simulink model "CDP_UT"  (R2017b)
settings: Solver=FixedStepDiscrete  StartTime=0.0  StopTime=10.0  FixedStep=0.01  RelTol=1e-3  EnableMultiTasking=on
undefined symbols (not defined in the file): ASWTYPE_FALSE, ASWTYPE_TRUE, CaCDP_CellTempNTCVoltTable_mV, CaCDP_CellTempTable_C, CaCDP_CMUPCBTempNTCVoltTable_mV, CaCDP_CMUPCBTempTable_C, CbCDP_DiffBusbarTempStateCheck_flg, CbCDP_DiffCellTempStateCheck_flg, CbCDP_DiffCellVoltStateCheck_flg, CbCDP_IgnorUpdateVld_flg, CbCDP_MaxBusbarTempStateCheck_flg, CbCDP_MaxCellTempStateCheck_flg, CbCDP_MaxCellVoltStateCheck_flg, CbCDP_MinBusbarTempStateCheck_flg, CbCDP_MinCellTempStateCheck_flg, CbCDP_MinCellVoltStateCheck_flg, CcCDP_AFETempConfig_numb, CcCDP_AFETempFltThd_C, CcCDP_AFETempFltThdHys_C, CcCDP_BusbarTempRngFltHiThrd_C, CcCDP_BusbarTempRngFltLowThrd_C, CcCDP_CellDiffFltLevel1_mV, CcCDP_CellDiffFltLevel2_mV, CcCDP_CellDiffFltLevel3_mV, CcCDP_CellTempLowerLimit_C, CcCDP_CellTempRngFltHiThrd_C, CcCDP_CellTempRngFltLowThrd_C, CcCDP_CellTempUpperLimit_C, CcCDP_CellVoltConfig_numb, CcCDP_CellVoltLowerLimit_mV, CcCDP_CellVoltRngHiThrd_mV, CcCDP_CellVoltRngLowThrd_mV, CcCDP_CellVoltUpdateThrd_numb, CcCDP_CellVoltUpperLimit_mV, CcCDP_ChrgMaxCellTempFltLv1Thrd_C, CcCDP_ChrgMaxCellTempFltLv2Thrd_C, CcCDP_ChrgMaxCellTempFltLv3Thrd_C, CcCDP_ChrgMaxCellTempReturnDiff_C, CcCDP_ChrgMinCellTempFltLv1Thrd_C, CcCDP_ChrgMinCellTempFltLv2Thrd_C, CcCDP_ChrgMinCellTempFltLv3Thrd_C, CcCDP_ChrgMinCellTempReturnDiff_C, CcCDP_CMUPCBTempConfig_numb, CcCDP_CMUPCBTempFltThd_C, CcCDP_CMUPCBTempFltThdHys_C, CcCDP_DiffBusbarTempFltLevel1Thrd_C, CcCDP_DiffBusbarTempFltLevel2Thrd_C, CcCDP_DiffBusbarTempReturnDifference_C, CcCDP_DiffCellTempFltLevel1Thrd_C, CcCDP_DiffCellTempFltLevel2Thrd_C, CcCDP_DiffCellTempReturnDifference_C, CcCDP_DiffCellVoltReturnDifference_mV, CcCDP_DiffVoltCheckMaxCellTempCondition_C, CcCDP_DiffVoltCheckMaxCellVoltCondition_mV, CcCDP_DiffVoltCheckMinCellTempCondition_C, CcCDP_DiffVoltCheckMinCellVoltCondition_mV, CcCDP_DiffVoltCheckPackCurrCondition_A, CcCDP_MaxAFETempIniVal_C, CcCDP_MaxBusbarTempFltLevel1Thrd_C, CcCDP_MaxBusbarTempFltLevel2Thrd_C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
libraries: AIWAYS_Powertrain_BMS_lib x148, simulink x8
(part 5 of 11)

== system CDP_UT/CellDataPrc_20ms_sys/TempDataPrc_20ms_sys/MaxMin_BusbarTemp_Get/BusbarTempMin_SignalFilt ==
  GeUDS_CapSel_enum : Inport
  LbCDP_AnyBusbarTempVld_flg : Inport  Port=2
  LcCDP_MinBusbarTemp_C : Inport  Port=3
  LcCDP_MinBusbarTempNumb_numb : Inport  Port=4
  1D_Config_Word : AIWAYS_Powertrain_BMS_lib/Signals/1D_Config_Word  Default_CalPar_Name=CcCDP_CATL203MaxCellTempFilCfig_numb  CATL153Ah_CalPar_Name=CcCDP_CATL177MaxCellTempFilCfig_numb  CATL180Ah_CalPar_Name=CcCDP_CATL177MaxCellTempFilCfig_numb  CATL177Ah_CalPar_Name=CcCDP_CATL177MaxCellTempFilCfig_numb  CATL203Ah_CalPar_Name=CcCDP_CATL203MaxCellTempFilCfig_numb  CATL51Ah_CalPar_Name=CcCDP_CATL177MaxCellTempFilCfig_numb  CATL132Ah_CalPar_Name=CcCDP_CATL177MaxCellTempFilCfig_numb  XWD75Ah_CalPar_Name=CcCDP_CATL177MaxCellTempFilCfig_numb  TFE177Ah_CalPar_Name=CcCDP_CATL177MaxCellTempFilCfig_numb  CATLCTP248Ah_CalPar_Name=CcCDP_CATL177MaxCellTempFilCfig_numb
  InputValueCalc : Stateflow chart  TreatAsAtomicUnit=on
  MaxValue_sort : Stateflow chart  TreatAsAtomicUnit=on
  SignalDelay1 : Subsystem  Commented=on
  Unit Delay21 : UnitDelay  SampleTime=-1  StateName=StateName
  ValueCalc : Subsystem
  ValueIndexCalc : Subsystem
  GcCDP_MinBusbarTemp_C : Outport
  GcCDP_MinBusbarTempNumb_numb : Outport  Port=2
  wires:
  LbCDP_AnyBusbarTempVld_flg/1 -> InputValueCalc/2(Rige), ValueIndexCalc/3(LbCDP_AnyBusbarTempVld_flg)
  GeUDS_CapSel_enum/1 -> 1D_Config_Word/1
  InputValueCalc/1(Output_Value) -> Unit Delay21/1, MaxValue_sort/1(Input_Value)
  1D_Config_Word/1 -> ValueCalc/3(CcCDP_CellTempFilConfig_numb), MaxValue_sort/2(Input_dim)
  ValueCalc/1(GcCDP_MinBusbarTemp_C) -> GcCDP_MinBusbarTemp_C/1
  ValueIndexCalc/1(GcCDP_MinBusbarTempNumb_numb) -> GcCDP_MinBusbarTempNumb_numb/1
  LcCDP_MinBusbarTempNumb_numb/1 -> ValueIndexCalc/2(LcCDP_MinBusbarTempNumb_numb)
  LcCDP_MinBusbarTemp_C/1 -> InputValueCalc/1(Input_Value)
  Unit Delay21/1 -> InputValueCalc/3(Old_Value)
  MaxValue_sort/1(Output_Value) -> ValueCalc/1(Output_Value)
  MaxValue_sort/2(Output_index) -> ValueCalc/2(Output_index)
  ValueCalc/2(Output_index1) -> ValueIndexCalc/1(Output_index1)

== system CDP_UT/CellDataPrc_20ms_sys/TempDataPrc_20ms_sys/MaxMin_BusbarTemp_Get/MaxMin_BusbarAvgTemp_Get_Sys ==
  LaCDP_BusbarTemp_C : Inport
  GcUDS_BusbarTempNumb_numb : Inport  Port=2
  Enable : EnablePort  StatesWhenEnabling=reset
  Divide1 : Product  Inputs=*/  OutDataTypeStr=single
  MinBusbarTemp_ForIterator : Subsystem  TreatAsAtomicUnit=on
  OverWrite1 : AIWAYS_Powertrain_BMS_lib/Signals/OverWrite  OverWrite_Value=CcCDP_AvgBusbarTempOvr_C  OverWrite_flag=CbCDP_AvgBusbarTempOvrSwt_flg
  GcCDP_AvgBusbarTemp_C : Outport
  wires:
  GcUDS_BusbarTempNumb_numb/1 -> Divide1/2, MinBusbarTemp_ForIterator/2(GcUDS_BusbarTempNumb_numb)
  MinBusbarTemp_ForIterator/1(LcCDP_SumBusbarTemp_C) -> Divide1/1
  Divide1/1 -> OverWrite1/1
  OverWrite1/1 -> GcCDP_AvgBusbarTemp_C/1  "GcCDP_AvgBusbarTemp_C"
  LaCDP_BusbarTemp_C/1 -> MinBusbarTemp_ForIterator/1(LaCDP_BusbarTemp_C)

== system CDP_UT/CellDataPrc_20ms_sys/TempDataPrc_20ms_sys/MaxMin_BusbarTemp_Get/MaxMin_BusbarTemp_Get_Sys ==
  LaCDP_BusbarTempVld_flg : Inport
  LaCDP_BusbarTemp_C : Inport  Port=2
  GcUDS_BusbarTempNumb_numb : Inport  Port=3
  GaISP_BusbarTempUpdCnt_numb : Inport  Port=4
  Enable : EnablePort  StatesWhenEnabling=reset
  Comparison4 : RelationalOperator  Operator===  OutDataTypeStr=boolean
  Constant1 : Constant  Value=CDP_CONST0_NUMB
  Constant2 : Constant  Value=CbCDP_IgnorUpdateVld_flg
  Logical : Logic  OutDataTypeStr=boolean
  MinBusbarTemp_ForIterator : Subsystem  TreatAsAtomicUnit=on
  Switch : Switch  Criteria=u2 ~= 0  Threshold=1  RndMeth=Zero
  LcCDP_MaxBusbarTemp_C : Outport
  LcCDP_MaxBusbarTempNumb_numb : Outport  Port=2
  LcCDP_MinBusbarTemp_C : Outport  Port=3
  LcCDP_MinBusbarTempNumb_numb : Outport  Port=4
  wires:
  MinBusbarTemp_ForIterator/3(LcCDP_MaxBusbarTempNumb_numb) -> LcCDP_MaxBusbarTempNumb_numb/1  "LcCDP_MaxBusbarTempNumb_numb"
  MinBusbarTemp_ForIterator/4(LcCDP_MaxBusbarTemp_C) -> LcCDP_MaxBusbarTemp_C/1  "LcCDP_MaxBusbarTemp_C"
  MinBusbarTemp_ForIterator/1(LcCDP_MinBusbarTemp_C) -> LcCDP_MinBusbarTemp_C/1  "LcCDP_MinBusbarTemp_C"
  MinBusbarTemp_ForIterator/2(LcCDP_MinBusbarTempNumb_numb) -> LcCDP_MinBusbarTempNumb_numb/1  "LcCDP_MinBusbarTempNumb_numb"
  LaCDP_BusbarTemp_C/1 -> MinBusbarTemp_ForIterator/1(LaCDP_BusbarTemp_C)
  GcUDS_BusbarTempNumb_numb/1 -> MinBusbarTemp_ForIterator/3(GcUDS_BusbarTempNumb_numb)
  Comparison4/1 -> Logical/2
  GaISP_BusbarTempUpdCnt_numb/1 -> Comparison4/1
  LaCDP_BusbarTempVld_flg/1 -> Logical/1, Switch/1
  Logical/1 -> Switch/3
  Constant1/1 -> Comparison4/2
  Constant2/1 -> Switch/2
  Switch/1 -> MinBusbarTemp_ForIterator/2(LaCDP_BusbarTempVld_flg)

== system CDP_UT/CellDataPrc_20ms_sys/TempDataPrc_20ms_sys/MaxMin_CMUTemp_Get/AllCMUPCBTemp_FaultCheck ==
  GaCDP_CMUPCBTempVld_flg : Inport
  CMUTempVld : Subsystem
  Constant4 : Constant  Value=CcCDP_CMUPCBTempConfig_numb
  LbCDP_AnyCMUTempVld_flg : Outport
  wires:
  GaCDP_CMUPCBTempVld_flg/1 -> CMUTempVld/1(GaCDP_CMUPCBTempVld_flg)
  Constant4/1 -> CMUTempVld/2(CcCDP_CMUTempConfig_numb)
  CMUTempVld/1(LbCDP_AnyCMUTempVld_flg) -> LbCDP_AnyCMUTempVld_flg/1

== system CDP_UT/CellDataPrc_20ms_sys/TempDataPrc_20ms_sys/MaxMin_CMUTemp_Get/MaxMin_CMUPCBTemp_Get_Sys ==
  GaCDP_CMUPCBTempVld_flg : Inport
  GaCDP_CMUPCBTemp_C : Inport  Port=2
  Enable : EnablePort  StatesWhenEnabling=reset
  CDP_GcCDP_MaxCMUPCBTempNumb_numb : AIWAYS_Powertrain_BMS_lib/Signals/OverWrite  OverWrite_Value=CcCDP_MaxCMUPCBTempNumbOvr_numb  OverWrite_flag=CbCDP_MaxCMUPCBTempNumbOvrSwt_flg
  CDP_GcCDP_MaxCMUPCBTemp_C : AIWAYS_Powertrain_BMS_lib/Signals/OverWrite  OverWrite_Value=CcCDP_MaxCMUPCBTempOvr_C  OverWrite_flag=CbCDP_MaxCMUPCBTempOvrSwt_flg
  CDP_GcCDP_MinCMUPCBTempNumb_numb : AIWAYS_Powertrain_BMS_lib/Signals/OverWrite  OverWrite_Value=CcCDP_MinCMUPCBTempNumbOvr_numb  OverWrite_flag=CbCDP_MinCMUPCBTempNumbOvrSwt_flg
  CDP_GcCDP_MinCMUPCBTemp_C : AIWAYS_Powertrain_BMS_lib/Signals/OverWrite  OverWrite_Value=CcCDP_MinCMUPCBTempOvr_C  OverWrite_flag=CbCDP_MinCMUPCBTempOvrSwt_flg
  Constant3 : Constant  Value=CcCDP_CMUPCBTempConfig_numb
  MinCMUTemp_ForIterator : Subsystem  TreatAsAtomicUnit=on
  GcCDP_MaxCMUPCBTemp_C : Outport
  GcCDP_MaxCMUPCBTempNumb_numb : Outport  Port=2
  GcCDP_MinCMUPCBTemp_C : Outport  Port=3
  GcCDP_MinCMUPCBTempNumb_numb : Outport  Port=4
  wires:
  Constant3/1 -> MinCMUTemp_ForIterator/3(CcCDP_CMUPCBTempConfig_numb)  "CcCDP_CMUPCBTempConfig_numb"
  GaCDP_CMUPCBTemp_C/1 -> MinCMUTemp_ForIterator/1(GaCDP_CMUPCBTemp_C)
  MinCMUTemp_ForIterator/1(LcCDP_MinCMUPCBTemp_C) -> CDP_GcCDP_MinCMUPCBTemp_C/1
  MinCMUTemp_ForIterator/2(LcCDP_MinCMUPCBTempNumb_numb) -> CDP_GcCDP_MinCMUPCBTempNumb_numb/1
  GaCDP_CMUPCBTempVld_flg/1 -> MinCMUTemp_ForIterator/2(GaCDP_CMUPCBTempVld_flg)
  CDP_GcCDP_MinCMUPCBTempNumb_numb/1 -> GcCDP_MinCMUPCBTempNumb_numb/1  "GcCDP_MinCMUPCBTempNumb_numb"
  CDP_GcCDP_MinCMUPCBTemp_C/1 -> GcCDP_MinCMUPCBTemp_C/1  "GcCDP_MinCMUPCBTemp_C"
  CDP_GcCDP_MaxCMUPCBTempNumb_numb/1 -> GcCDP_MaxCMUPCBTempNumb_numb/1  "GcCDP_MaxCMUPCBTempNumb_numb"
  CDP_GcCDP_MaxCMUPCBTemp_C/1 -> GcCDP_MaxCMUPCBTemp_C/1  "GcCDP_MaxCMUPCBTemp_C"
  MinCMUTemp_ForIterator/3(LcCDP_MaxCMUPCBTempNumb_numb) -> CDP_GcCDP_MaxCMUPCBTempNumb_numb/1
  MinCMUTemp_ForIterator/4(LcCDP_MaxCMUPCBTemp_C) -> CDP_GcCDP_MaxCMUPCBTemp_C/1

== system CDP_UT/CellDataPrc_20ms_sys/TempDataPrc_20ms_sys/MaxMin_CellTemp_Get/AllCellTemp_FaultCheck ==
  GaCDP_CellTempVld_flg : Inport
  GcUDS_CellTempNumb_numb : Inport  Port=2
  GaISP_CellTempUpdCnt_numb : Inport  Port=3
  CellTempVld : Subsystem
  Comparison4 : RelationalOperator  Operator===  OutDataTypeStr=boolean
  Constant1 : Constant  Value=CDP_CONST0_NUMB
  Constant2 : Constant  Value=CbCDP_IgnorUpdateVld_flg
  Logical : Logic  OutDataTypeStr=boolean
  OverWrite : AIWAYS_Powertrain_BMS_lib/Signals/OverWrite  OverWrite_Value=CbCDP_AllCellTempVldOvr_flg  OverWrite_flag=CbCDP_AllCellTempVldOvrSwt_flg
  Switch : Switch  Criteria=u2 ~= 0  Threshold=1  RndMeth=Zero
  GbCDP_AllCellTempVld_flg : Outport
  LbCDP_AnyCellTempVld_flg : Outport  Port=2
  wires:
  CellTempVld/1(LbCDP_CellTempVld_flg) -> OverWrite/1
  OverWrite/1 -> GbCDP_AllCellTempVld_flg/1  "GbCDP_AllCellTempVld_flg"
  GcUDS_CellTempNumb_numb/1 -> CellTempVld/2(GcUDS_CellTempNumb_numb)
  CellTempVld/2(LbCDP_AnyCellTempVld_flg) -> LbCDP_AnyCellTempVld_flg/1
  Switch/1 -> CellTempVld/1(GaCDP_CellTempVld_flg)
  GaCDP_CellTempVld_flg/1 -> Switch/1, Logical/1
  GaISP_CellTempUpdCnt_numb/1 -> Comparison4/1
  Constant2/1 -> Switch/2
  Constant1/1 -> Comparison4/2
  Logical/1 -> Switch/3
  Comparison4/1 -> Logical/2

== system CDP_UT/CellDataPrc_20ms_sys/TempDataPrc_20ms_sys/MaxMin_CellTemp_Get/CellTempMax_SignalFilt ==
  LcCDP_MaxCellTemp_C : Inport
  LcCDP_MaxCellTempNumb_numb : Inport  Port=2
  LbCDP_AnyCellTempVld_flg : Inport  Port=3
  GeUDS_CapSel_enum : Inport  Port=4
  1D_Config_Word : AIWAYS_Powertrain_BMS_lib/Signals/1D_Config_Word  Default_CalPar_Name=CcCDP_CATL203MaxCellTempFilCfig_numb  CATL153Ah_CalPar_Name=CcCDP_CATL177MaxCellTempFilCfig_numb  CATL180Ah_CalPar_Name=CcCDP_CATL177MaxCellTempFilCfig_numb  CATL177Ah_CalPar_Name=CcCDP_CATL177MaxCellTempFilCfig_numb  CATL203Ah_CalPar_Name=CcCDP_CATL203MaxCellTempFilCfig_numb  CATL51Ah_CalPar_Name=CcCDP_CATL177MaxCellTempFilCfig_numb  CATL132Ah_CalPar_Name=CcCDP_CATL177MaxCellTempFilCfig_numb  XWD75Ah_CalPar_Name=CcCDP_CATL177MaxCellTempFilCfig_numb  TFE177Ah_CalPar_Name=CcCDP_CATL177MaxCellTempFilCfig_numb  CATLCTP248Ah_CalPar_Name=CcCDP_CATL177MaxCellTempFilCfig_numb
  InputValueCalc : Stateflow chart  TreatAsAtomicUnit=on
  MaxValue_sort : Stateflow chart  TreatAsAtomicUnit=on
  SignalDelay1 : Subsystem  Commented=on
  Unit Delay21 : UnitDelay  SampleTime=-1  StateName=StateName
  ValueCalc : Subsystem
  ValueIndexCalc : Subsystem
  GcCDP_MaxCellTemp_C : Outport
  GcCDP_MaxCellTempNumb_numb : Outport  Port=2
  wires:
  ValueCalc/2(Output_index1) -> ValueIndexCalc/1(Output_index1)
  MaxValue_sort/2(Output_index) -> ValueCalc/2(Output_index)
  MaxValue_sort/1(Output_Value) -> ValueCalc/1(Output_Value)
  Unit Delay21/1 -> InputValueCalc/3(Old_Value)
  LcCDP_MaxCellTemp_C/1 -> InputValueCalc/1(Input_Value)
  LcCDP_MaxCellTempNumb_numb/1 -> ValueIndexCalc/2(LcCDP_MaxCellTempNumb_numb)
  ValueIndexCalc/1(GcCDP_MaxCellTempNumb_numb) -> GcCDP_MaxCellTempNumb_numb/1
  ValueCalc/1(GcCDP_MaxCellTemp_C) -> GcCDP_MaxCellTemp_C/1
  1D_Config_Word/1 -> MaxValue_sort/2(Input_dim), ValueCalc/3(CcCDP_CellTempFilConfig_numb)
  InputValueCalc/1(Output_Value) -> MaxValue_sort/1(Input_Value), Unit Delay21/1
  GeUDS_CapSel_enum/1 -> 1D_Config_Word/1
  LbCDP_AnyCellTempVld_flg/1 -> ValueIndexCalc/3(LbCDP_AnyCellTempVld_flg), InputValueCalc/2(Rige)

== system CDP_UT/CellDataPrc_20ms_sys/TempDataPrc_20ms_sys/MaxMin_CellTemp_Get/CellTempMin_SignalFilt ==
  GeUDS_CapSel_enum : Inport
  LbCDP_AnyCellTempVld_flg : Inport  Port=2
  LcCDP_MinCellTemp_C : Inport  Port=3
  LcCDP_MinCellTempNumb_numb : Inport  Port=4
  1D_Config_Word : AIWAYS_Powertrain_BMS_lib/Signals/1D_Config_Word  Default_CalPar_Name=CcCDP_CATL203MaxCellTempFilCfig_numb  CATL153Ah_CalPar_Name=CcCDP_CATL177MaxCellTempFilCfig_numb  CATL180Ah_CalPar_Name=CcCDP_CATL177MaxCellTempFilCfig_numb  CATL177Ah_CalPar_Name=CcCDP_CATL177MaxCellTempFilCfig_numb  CATL203Ah_CalPar_Name=CcCDP_CATL203MaxCellTempFilCfig_numb  CATL51Ah_CalPar_Name=CcCDP_CATL177MaxCellTempFilCfig_numb  CATL132Ah_CalPar_Name=CcCDP_CATL177MaxCellTempFilCfig_numb  XWD75Ah_CalPar_Name=CcCDP_CATL177MaxCellTempFilCfig_numb  TFE177Ah_CalPar_Name=CcCDP_CATL177MaxCellTempFilCfig_numb  CATLCTP248Ah_CalPar_Name=CcCDP_CATL177MaxCellTempFilCfig_numb
  InputValueCalc : Stateflow chart  TreatAsAtomicUnit=on
  MaxValue_sort : Stateflow chart  TreatAsAtomicUnit=on
  SignalDelay1 : Subsystem  Commented=on
  Unit Delay21 : UnitDelay  SampleTime=-1  StateName=StateName
  ValueCalc : Subsystem
  ValueIndexCalc : Subsystem
  GcCDP_MinCellTemp_C : Outport
  GcCDP_MinCellTempNumb_numb : Outport  Port=2
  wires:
  LbCDP_AnyCellTempVld_flg/1 -> InputValueCalc/2(Rige), ValueIndexCalc/3(LbCDP_AnyCellTempVld_flg)
  GeUDS_CapSel_enum/1 -> 1D_Config_Word/1
  InputValueCalc/1(Output_Value) -> Unit Delay21/1, MaxValue_sort/1(Input_Value)
  1D_Config_Word/1 -> ValueCalc/3(CcCDP_CellTempFilConfig_numb), MaxValue_sort/2(Input_dim)
  ValueCalc/1(GcCDP_MinCellTemp_C) -> GcCDP_MinCellTemp_C/1
  ValueIndexCalc/1(GcCDP_MinCellTempNumb_numb) -> GcCDP_MinCellTempNumb_numb/1
  LcCDP_MinCellTempNumb_numb/1 -> ValueIndexCalc/2(LcCDP_MinCellTempNumb_numb)
  LcCDP_MinCellTemp_C/1 -> InputValueCalc/1(Input_Value)
  Unit Delay21/1 -> InputValueCalc/3(Old_Value)
  MaxValue_sort/1(Output_Value) -> ValueCalc/1(Output_Value)
  MaxValue_sort/2(Output_index) -> ValueCalc/2(Output_index)
  ValueCalc/2(Output_index1) -> ValueIndexCalc/1(Output_index1)

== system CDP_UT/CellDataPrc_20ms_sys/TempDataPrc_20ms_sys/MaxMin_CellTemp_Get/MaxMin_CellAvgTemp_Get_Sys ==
  LaCDP_CellTemp_C : Inport
  GcUDS_CellTempNumb_numb : Inport  Port=2
  Enable : EnablePort  StatesWhenEnabling=reset
  Divide1 : Product  Inputs=*/  OutDataTypeStr=single
  MinCellTemp_ForIterator : Subsystem  TreatAsAtomicUnit=on
  OverWrite1 : AIWAYS_Powertrain_BMS_lib/Signals/OverWrite  OverWrite_Value=CcCDP_AvgCellTempOvr_C  OverWrite_flag=CbCDP_AvgCellTempOvrSwt_flg
  GcCDP_AvgCellTemp_C : Outport
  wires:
  LaCDP_CellTemp_C/1 -> MinCellTemp_ForIterator/1(LaCDP_CellTemp_C)
  OverWrite1/1 -> GcCDP_AvgCellTemp_C/1  "GcCDP_AvgCellTemp_C"
  Divide1/1 -> OverWrite1/1
  MinCellTemp_ForIterator/1(LcCDP_SumCellTemp_C) -> Divide1/1
  GcUDS_CellTempNumb_numb/1 -> MinCellTemp_ForIterator/2(GcUDS_CellTempNumb_numb), Divide1/2

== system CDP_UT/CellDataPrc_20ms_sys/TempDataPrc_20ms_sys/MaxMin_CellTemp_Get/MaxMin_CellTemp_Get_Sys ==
  GaCDP_CellTempVld_flg : Inport
  LaCDP_CellTemp_C : Inport  Port=2
  GcUDS_CellTempNumb_numb : Inport  Port=3
  GaISP_CellTempUpdCnt_numb : Inport  Port=4
  Enable : EnablePort  StatesWhenEnabling=reset
  Comparison4 : RelationalOperator  Operator===  OutDataTypeStr=boolean
  Constant1 : Constant  Value=CDP_CONST0_NUMB
  Constant2 : Constant  Value=CbCDP_IgnorUpdateVld_flg
  Logical : Logic  OutDataTypeStr=boolean
  MinCellTemp_ForIterator : Subsystem  TreatAsAtomicUnit=on
  Switch : Switch  Criteria=u2 ~= 0  Threshold=1  RndMeth=Zero
  LcCDP_MaxCellTemp_C : Outport
  LcCDP_MaxCellTempNumb_numb : Outport  Port=2
  LcCDP_MinCellTemp_C : Outport  Port=3
  LcCDP_MinCellTempNumb_numb : Outport  Port=4
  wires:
  MinCellTemp_ForIterator/1(LcCDP_MinCellTemp_C) -> LcCDP_MinCellTemp_C/1  "LcCDP_MinCellTemp_C"
  MinCellTemp_ForIterator/2(LcCDP_MinCellTempNumb_numb) -> LcCDP_MinCellTempNumb_numb/1  "LcCDP_MinCellTempNumb_numb"
  MinCellTemp_ForIterator/3(LcCDP_MaxCellTempNumb_numb) -> LcCDP_MaxCellTempNumb_numb/1  "LcCDP_MaxCellTempNumb_numb"
  MinCellTemp_ForIterator/4(LcCDP_MaxCellTemp_C) -> LcCDP_MaxCellTemp_C/1  "LcCDP_MaxCellTemp_C"
  GcUDS_CellTempNumb_numb/1 -> MinCellTemp_ForIterator/3(GcUDS_CellTempNumb_numb)
  GaCDP_CellTempVld_flg/1 -> Switch/1, Logical/1
  Comparison4/1 -> Logical/2
  Logical/1 -> Switch/3
  Constant1/1 -> Comparison4/2
  GaISP_CellTempUpdCnt_numb/1 -> Comparison4/1
  Constant2/1 -> Switch/2
  LaCDP_CellTemp_C/1 -> MinCellTemp_ForIterator/1(LaCDP_CellTemp_C)
  Switch/1 -> MinCellTemp_ForIterator/2(GaCDP_CellTempVld_flg)

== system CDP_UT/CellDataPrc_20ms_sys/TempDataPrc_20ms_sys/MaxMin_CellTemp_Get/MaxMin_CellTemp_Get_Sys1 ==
  GaCDP_CellTempVld_flg : Inport
  GaCDP_CellTemp_C : Inport  Port=2
  GcUDS_CellTempNumb_numb : Inport  Port=3
  Enable : EnablePort  StatesWhenEnabling=reset
  MinCellTemp_ForIterator : Subsystem  TreatAsAtomicUnit=on
  OverWrite : AIWAYS_Powertrain_BMS_lib/Signals/OverWrite  OverWrite_Value=CcCDP_MinCellTempOvr_C  OverWrite_flag=CbCDP_MinCellTempOvrSwt_flg
  OverWrite1 : AIWAYS_Powertrain_BMS_lib/Signals/OverWrite  OverWrite_Value=CcCDP_MinCellTempNumbOvr_numb  OverWrite_flag=CbCDP_MinCellTempNumbOvrSwt_flg
  OverWrite2 : AIWAYS_Powertrain_BMS_lib/Signals/OverWrite  OverWrite_Value=CcCDP_MaxCellTempOvr_C  OverWrite_flag=CbCDP_MaxCellTempOvrSwt_flg
  OverWrite3 : AIWAYS_Powertrain_BMS_lib/Signals/OverWrite  OverWrite_Value=CcCDP_MaxCellTempNumbOvr_numb  OverWrite_flag=CbCDP_MaxCellTempNumbOvrSwt_flg
  GcCDP_MaxCellTemp_C : Outport
  GcCDP_MaxCellTempNumb_numb : Outport  Port=2
  GcCDP_MinCellTemp_C : Outport  Port=3
  GcCDP_MinCellTempNumb_numb : Outport  Port=4
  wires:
  GaCDP_CellTemp_C/1 -> MinCellTemp_ForIterator/1(GaCDP_CellTemp_C)
  OverWrite1/1 -> GcCDP_MinCellTempNumb_numb/1  "GcCDP_MinCellTempNumb_numb"
  OverWrite/1 -> GcCDP_MinCellTemp_C/1  "GcCDP_MinCellTemp_C"
  OverWrite2/1 -> GcCDP_MaxCellTemp_C/1  "GcCDP_MaxCellTemp_C"
  OverWrite3/1 -> GcCDP_MaxCellTempNumb_numb/1  "GcCDP_MaxCellTempNumb_numb"
  MinCellTemp_ForIterator/1(LcCDP_MinCellTemp_C) -> OverWrite/1
  MinCellTemp_ForIterator/2(LcCDP_MinCellTempNumb_numb) -> OverWrite1/1
  MinCellTemp_ForIterator/3(LcCDP_MaxCellTempNumb_numb) -> OverWrite3/1
  MinCellTemp_ForIterator/4(LcCDP_MaxCellTemp_C) -> OverWrite2/1
  GaCDP_CellTempVld_flg/1 -> MinCellTemp_ForIterator/2(GaCDP_CellTempVld_flg)
  GcUDS_CellTempNumb_numb/1 -> MinCellTemp_ForIterator/3(GcUDS_CellTempNumb_numb)

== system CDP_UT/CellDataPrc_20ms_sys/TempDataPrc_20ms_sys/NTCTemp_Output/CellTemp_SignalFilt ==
  GcUDS_CellTempNumb_numb : Inport
  GeUDS_CapSel_enum : Inport  Port=2
  LaCDP_CellTempUpdateVld_flg : Inport  Port=3
  LaCDP_CellTemp_C : Inport  Port=4
  1D_Config_Word : AIWAYS_Powertrain_BMS_lib/Signals/1D_Config_Word  Default_CalPar_Name=CcCDP_CATL203CellTempFilCfig_numb  CATL153Ah_CalPar_Name=CcCDP_CATL177CellTempFilCfig_numb  CATL180Ah_CalPar_Name=CcCDP_CATL177CellTempFilCfig_numb  CATL177Ah_CalPar_Name=CcCDP_CATL177CellTempFilCfig_numb  CATL203Ah_CalPar_Name=CcCDP_CATL203CellTempFilCfig_numb  CATL51Ah_CalPar_Name=CcCDP_CATL177CellTempFilCfig_numb  CATL132Ah_CalPar_Name=CcCDP_CATL177CellTempFilCfig_numb  XWD75Ah_CalPar_Name=CcCDP_CATL177CellTempFilCfig_numb  TFE177Ah_CalPar_Name=CcCDP_CATL177CellTempFilCfig_numb  CATLCTP248Ah_CalPar_Name=CcCDP_CATL177CellTempFilCfig_numb
  Comparison1 : RelationalOperator  Operator===  OutDataTypeStr=boolean
  Constant6 : Constant  Value=ASWTYPE_FALSE
  InputValueCalc : Stateflow chart  TreatAsAtomicUnit=on
  MaxValue_sort : Stateflow chart  TreatAsAtomicUnit=on
  SignalDelay1 : Subsystem  Commented=on
  Terminator : Terminator
  Unit Delay21 : UnitDelay  SampleTime=-1  StateName=StateName
  GaCDP_CellTemp_C : Outport
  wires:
  Unit Delay21/1 -> InputValueCalc/4(Old_Value)
  LaCDP_CellTemp_C/1 -> InputValueCalc/1(Input_Value)
  1D_Config_Word/1 -> MaxValue_sort/2(Input_dim)
  InputValueCalc/1(Output_Value) -> Unit Delay21/1, MaxValue_sort/1(Input_Value)
  GeUDS_CapSel_enum/1 -> 1D_Config_Word/1
  LaCDP_CellTempUpdateVld_flg/1 -> Comparison1/1
  MaxValue_sort/1(Output_Value) -> Terminator/1
  GcUDS_CellTempNumb_numb/1 -> MaxValue_sort/3(Input_num), InputValueCalc/3(Input_num)
  MaxValue_sort/2(TargetOutput_Value) -> GaCDP_CellTemp_C/1  "GaCDP_CellTemp_C"
  Constant6/1 -> Comparison1/2
  Comparison1/1 -> InputValueCalc/2(Update)  "LaCDP_CellTempUpdateVld_flg"

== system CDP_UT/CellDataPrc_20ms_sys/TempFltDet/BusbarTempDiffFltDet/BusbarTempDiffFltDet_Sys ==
  LbCDP_DiffBusbarTempChkCond_flg : Inport
  GcCDP_MaxBusbarTemp_C : Inport  Port=2
  GcCDP_MinBusbarTemp_C : Inport  Port=3
  LbCDP_BusbarTempRngHiFlt_flg : Inport  Port=4
  LbCDP_BusbarTempRngLowFlt_flg : Inport  Port=5
  Add : Sum  Inputs=+-  OutDataTypeStr=Inherit: Inherit via back propagation
  Bus Creator : BusCreator  Inputs=4
  Bus Selector : BusSelector  OutputSignals=LcCDP_DiffBusbarTemp_C,LbCDP_BusbarTempRngHiFlt_flg,LbCDP_BusbarTempRngLowFlt_flg,LbCDP_DiffBusbarTempChkCond_flg
  Bus Selector1 : BusSelector  OutputSignals=LbCDP_DiffBusbarTempChkCond_flg,LcCDP_DiffBusbarTemp_C,LbCDP_BusbarTempRngHiFlt_flg,LbCDP_BusbarTempRngLowFlt_flg
  BusbarTempDiffFltLv1Det : Subsystem
  BusbarTempDiffFltLv2Det : Subsystem
  GbCDP_BusbarTempDiffFltLv2_flg : Outport
  GbCDP_BusbarTempDiffFltLv1_flg : Outport  Port=2
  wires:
  Bus Selector1/4 -> BusbarTempDiffFltLv1Det/4(LbCDP_BusbarTempRngLowFlt_flg)  "<LbCDP_BusbarTempRngLowFlt_flg>"
  Bus Selector1/3 -> BusbarTempDiffFltLv1Det/3(LbCDP_BusbarTempRngHiFlt_flg)  "<LbCDP_BusbarTempRngHiFlt_flg>"
  Bus Selector1/2 -> BusbarTempDiffFltLv1Det/2(LcCDP_DiffBusbarTemp_C)  "<LcCDP_DiffBusbarTemp_C>"
  Bus Selector1/1 -> BusbarTempDiffFltLv1Det/1(LbCDP_DiffBusbarTempChkCond_flg)  "<LbCDP_DiffBusbarTempChkCond_flg>"
  Bus Selector/4 -> BusbarTempDiffFltLv2Det/4(LbCDP_DiffBusbarTempChkCond_flg)  "<LbCDP_DiffBusbarTempChkCond_flg>"
  LbCDP_DiffBusbarTempChkCond_flg/1 -> Bus Creator/4
  BusbarTempDiffFltLv1Det/1(GbCDP_BusbarTempDiffFltLv1_flg) -> GbCDP_BusbarTempDiffFltLv1_flg/1
  BusbarTempDiffFltLv2Det/1(GbCDP_BusbarTempDiffFltLv2_flg) -> GbCDP_BusbarTempDiffFltLv2_flg/1
  Bus Selector/3 -> BusbarTempDiffFltLv2Det/3(LbCDP_BusbarTempRngLowFlt_flg)  "<LbCDP_BusbarTempRngLowFlt_flg>"
  Bus Selector/2 -> BusbarTempDiffFltLv2Det/2(LbCDP_BusbarTempRngHiFlt_flg)  "<LbCDP_BusbarTempRngHiFlt_flg>"
  Bus Selector/1 -> BusbarTempDiffFltLv2Det/1(LcCDP_DiffBusbarTemp_C)  "<LcCDP_DiffBusbarTemp_C>"
  LbCDP_BusbarTempRngLowFlt_flg/1 -> Bus Creator/3
  LbCDP_BusbarTempRngHiFlt_flg/1 -> Bus Creator/2
  Bus Creator/1 -> Bus Selector/1, Bus Selector1/1
  GcCDP_MinBusbarTemp_C/1 -> Add/2
  GcCDP_MaxBusbarTemp_C/1 -> Add/1
  Add/1 -> Bus Creator/1  "LcCDP_DiffBusbarTemp_C"

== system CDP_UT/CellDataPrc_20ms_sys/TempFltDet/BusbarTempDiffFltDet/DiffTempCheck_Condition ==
  LbCDP_AnyBusbarTempVld_flg : Inport
  Constant : Constant  Value=ASWTYPE_TRUE
  Constant1 : Constant  Value=CbCDP_DiffBusbarTempStateCheck_flg
  Constant2 : Constant  Value=ASWTYPE_TRUE
  Logical Operator : Logic  AllPortsSameDT=off  OutDataTypeStr=boolean
  Relational Operator : RelationalOperator  Operator===  OutDataTypeStr=boolean
  Relational Operator1 : RelationalOperator  Operator===  OutDataTypeStr=boolean
  LbCDP_DiffBusbarTempChkCond_flg : Outport
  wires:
  Constant2/1 -> Relational Operator1/2
  Constant/1 -> Relational Operator/2
  Relational Operator/1 -> Logical Operator/1
  Relational Operator1/1 -> Logical Operator/2
  Logical Operator/1 -> LbCDP_DiffBusbarTempChkCond_flg/1  "LbCDP_DiffBusbarTempChkCond_flg"
  LbCDP_AnyBusbarTempVld_flg/1 -> Relational Operator/1
  Constant1/1 -> Relational Operator1/1

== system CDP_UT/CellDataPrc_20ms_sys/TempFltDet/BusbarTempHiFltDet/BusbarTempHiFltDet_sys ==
  LbCDP_MaxBusbarTempChkCond_flg : Inport
  GcCDP_MaxBusbarTemp_C : Inport  Port=2
  Bus Creator : BusCreator  Inputs=2
  Bus Selector : BusSelector  OutputSignals=LbCDP_MaxBusbarTempChkCond_flg,GcCDP_MaxBusbarTemp_C
  Bus Selector1 : BusSelector  OutputSignals=LbCDP_MaxBusbarTempChkCond_flg,GcCDP_MaxBusbarTemp_C
  Bus Selector2 : BusSelector  OutputSignals=LbCDP_MaxBusbarTempChkCond_flg,GcCDP_MaxBusbarTemp_C
  BusbarTempHiFltLv1Det : Subsystem
  BusbarTempHiFltLv2Det : Subsystem
  BusbarTempHiFltLv3Det : Subsystem
  GbCDP_BusbarTempHiFltLv3_flg : Outport
  GbCDP_BusbarTempHiFltLv2_flg : Outport  Port=2
  GbCDP_BusbarTempHiFltLv1_flg : Outport  Port=3
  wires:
  GcCDP_MaxBusbarTemp_C/1 -> Bus Creator/1
  Bus Creator/1 -> Bus Selector2/1, Bus Selector1/1, Bus Selector/1
  BusbarTempHiFltLv3Det/1(GbCDP_BusbarTempHiFltLv3_flg) -> GbCDP_BusbarTempHiFltLv3_flg/1
  LbCDP_MaxBusbarTempChkCond_flg/1 -> Bus Creator/2
  Bus Selector/1 -> BusbarTempHiFltLv3Det/1(LbCDP_MaxBusbarTempChkCond_flg)  "<LbCDP_MaxBusbarTempChkCond_flg>"
  Bus Selector/2 -> BusbarTempHiFltLv3Det/2(GcCDP_MaxBusbarTemp_C)  "<GcCDP_MaxBusbarTemp_C>"
  Bus Selector1/1 -> BusbarTempHiFltLv2Det/1(LbCDP_MaxBusbarTempChkCond_flg)  "<LbCDP_MaxBusbarTempChkCond_flg>"
  Bus Selector1/2 -> BusbarTempHiFltLv2Det/2(GcCDP_MaxBusbarTemp_C)  "<GcCDP_MaxBusbarTemp_C>"
  Bus Selector2/1 -> BusbarTempHiFltLv1Det/1(LbCDP_MaxBusbarTempChkCond_flg)  "<LbCDP_MaxBusbarTempChkCond_flg>"
  Bus Selector2/2 -> BusbarTempHiFltLv1Det/2(GcCDP_MaxBusbarTemp_C)  "<GcCDP_MaxBusbarTemp_C>"
  BusbarTempHiFltLv2Det/1(GbCDP_BusbarTempHiFltLv2_flg) -> GbCDP_BusbarTempHiFltLv2_flg/1
  BusbarTempHiFltLv1Det/1(GbCDP_BusbarTempHiFltLv1_flg) -> GbCDP_BusbarTempHiFltLv1_flg/1

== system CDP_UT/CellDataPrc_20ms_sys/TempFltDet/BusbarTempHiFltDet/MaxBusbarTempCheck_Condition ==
  LbCDP_AnyBusbarTempVld_flg : Inport
  Constant1 : Constant  Value=CbCDP_MaxBusbarTempStateCheck_flg
  Constant2 : Constant  Value=ASWTYPE_TRUE
  Constant3 : Constant  Value=ASWTYPE_TRUE
  Logical Operator : Logic  AllPortsSameDT=off  OutDataTypeStr=boolean
  Relational Operator1 : RelationalOperator  Operator===  OutDataTypeStr=boolean
  Relational Operator2 : RelationalOperator  Operator===  OutDataTypeStr=boolean
  LbCDP_MaxBusbarTempChkCond_flg : Outport
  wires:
  Constant1/1 -> Relational Operator1/1
  Logical Operator/1 -> LbCDP_MaxBusbarTempChkCond_flg/1  "LbCDP_MaxBusbarTempChkCond_flg"
  Constant2/1 -> Relational Operator1/2
  Relational Operator1/1 -> Logical Operator/2
  Constant3/1 -> Relational Operator2/2
  Relational Operator2/1 -> Logical Operator/1
  LbCDP_AnyBusbarTempVld_flg/1 -> Relational Operator2/1

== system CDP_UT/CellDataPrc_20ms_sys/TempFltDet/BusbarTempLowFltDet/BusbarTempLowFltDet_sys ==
  LbCDP_MinBusbarTempChkCond_flg : Inport
  GcCDP_MinBusbarTemp_C : Inport  Port=2
  Bus Creator : BusCreator  Inputs=2
  Bus Selector : BusSelector  OutputSignals=LbCDP_MinBusbarTempChkCond_flg,GcCDP_MinBusbarTemp_C
  Bus Selector1 : BusSelector  OutputSignals=LbCDP_MinBusbarTempChkCond_flg,GcCDP_MinBusbarTemp_C
  Bus Selector2 : BusSelector  OutputSignals=LbCDP_MinBusbarTempChkCond_flg,GcCDP_MinBusbarTemp_C
  BusbarTempLowFltLv1Det : Subsystem
  BusbarTempLowFltLv2Det : Subsystem
  BusbarTempLowFltLv3Det : Subsystem
  GbCDP_BusbarTempLowFltLv3_flg : Outport
  GbCDP_BusbarTempLowFltLv2_flg : Outport  Port=2
  GbCDP_BusbarTempLowFltLv1_flg : Outport  Port=3
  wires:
  GcCDP_MinBusbarTemp_C/1 -> Bus Creator/1
  Bus Creator/1 -> Bus Selector2/1, Bus Selector1/1, Bus Selector/1
  BusbarTempLowFltLv3Det/1(GbCDP_BusbarTempLowFltLv3_flg) -> GbCDP_BusbarTempLowFltLv3_flg/1
  LbCDP_MinBusbarTempChkCond_flg/1 -> Bus Creator/2
  Bus Selector/1 -> BusbarTempLowFltLv3Det/1(LbCDP_MinBusbarTempChkCond_flg)  "<LbCDP_MinBusbarTempChkCond_flg>"
  Bus Selector/2 -> BusbarTempLowFltLv3Det/2(GcCDP_MinBusbarTemp_C)  "<GcCDP_MinBusbarTemp_C>"
  Bus Selector1/1 -> BusbarTempLowFltLv2Det/1(LbCDP_MinBusbarTempChkCond_flg)  "<LbCDP_MinBusbarTempChkCond_flg>"
  Bus Selector1/2 -> BusbarTempLowFltLv2Det/2(GcCDP_MinBusbarTemp_C)  "<GcCDP_MinBusbarTemp_C>"
  Bus Selector2/1 -> BusbarTempLowFltLv1Det/1(LbCDP_MinBusbarTempChkCond_flg)  "<LbCDP_MinBusbarTempChkCond_flg>"
  Bus Selector2/2 -> BusbarTempLowFltLv1Det/2(GcCDP_MinBusbarTemp_C)  "<GcCDP_MinBusbarTemp_C>"
  BusbarTempLowFltLv2Det/1(GbCDP_BusbarTempLowFltLv2_flg) -> GbCDP_BusbarTempLowFltLv2_flg/1
  BusbarTempLowFltLv1Det/1(GbCDP_BusbarTempLowFltLv1_flg) -> GbCDP_BusbarTempLowFltLv1_flg/1

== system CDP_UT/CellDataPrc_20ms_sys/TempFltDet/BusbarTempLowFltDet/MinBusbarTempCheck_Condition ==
  LbCDP_AnyBusbarTempVld_flg : Inport
  Constant1 : Constant  Value=CbCDP_MinBusbarTempStateCheck_flg
  Constant2 : Constant  Value=ASWTYPE_TRUE
  Constant3 : Constant  Value=ASWTYPE_TRUE
  Logical Operator : Logic  AllPortsSameDT=off  OutDataTypeStr=boolean
  Relational Operator1 : RelationalOperator  Operator===  OutDataTypeStr=boolean
  Relational Operator2 : RelationalOperator  Operator===  OutDataTypeStr=boolean
  LbCDP_MinBusbarTempChkCond_flg : Outport
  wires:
  Constant1/1 -> Relational Operator1/1
  Logical Operator/1 -> LbCDP_MinBusbarTempChkCond_flg/1  "LbCDP_MinBusbarTempChkCond_flg"
  Constant2/1 -> Relational Operator1/2
  Relational Operator1/1 -> Logical Operator/2
  Constant3/1 -> Relational Operator2/2
  Relational Operator2/1 -> Logical Operator/1
  LbCDP_AnyBusbarTempVld_flg/1 -> Relational Operator2/1

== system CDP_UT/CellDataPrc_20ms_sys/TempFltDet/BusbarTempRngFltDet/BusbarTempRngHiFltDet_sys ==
  LbCDP_BusbarTempRngHiChk_flg : Inport
  GcCDP_MaxBusbarTemp_C : Inport  Port=2
  CDP_GbCDP_ChrgMaxCellVoltFltLv1_flg : AIWAYS_Powertrain_BMS_lib/Signals/OverWrite  OverWrite_Value=CbCDP_BusbarTempRngHiFltOvr_flg  OverWrite_flag=CbCDP_BusbarTempRngHiFltOvrSwt_flg
  Constant : Constant  Value=CcCDP_BusbarTempRngFltHiThrd_C
  Logical Operator1 : Logic  AllPortsSameDT=off  OutDataTypeStr=boolean
  Relational Operator : RelationalOperator  OutDataTypeStr=boolean
  LbCDP_BusbarTempRngHiFlt_flg : Outport
  GbCDP_BusbarTempRngHiFlt_flg : Outport  Port=2
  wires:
  LbCDP_BusbarTempRngHiChk_flg/1 -> Logical Operator1/1
  Relational Operator/1 -> Logical Operator1/2
  Logical Operator1/1 -> CDP_GbCDP_ChrgMaxCellVoltFltLv1_flg/1, LbCDP_BusbarTempRngHiFlt_flg/1  "LbCDP_BusbarTempRngHiFlt_flg"
  CDP_GbCDP_ChrgMaxCellVoltFltLv1_flg/1 -> GbCDP_BusbarTempRngHiFlt_flg/1  "GbCDP_BusbarTempRngHiFlt_flg"
  Constant/1 -> Relational Operator/2
  GcCDP_MaxBusbarTemp_C/1 -> Relational Operator/1

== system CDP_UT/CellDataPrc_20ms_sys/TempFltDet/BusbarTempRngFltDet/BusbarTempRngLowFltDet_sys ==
  LbCDP_BusbarTempRngLowChk_flg : Inport
  GcCDP_MinBusbarTemp_C : Inport  Port=2
  CDP_GbCDP_ChrgMaxCellVoltFltLv1_flg : AIWAYS_Powertrain_BMS_lib/Signals/OverWrite  OverWrite_Value=CbCDP_BusbarTempRngLowFltOvr_flg  OverWrite_flag=CbCDP_BusbarTempRngLowFltOvrSwt_flg
  Comparison3 : RelationalOperator  Operator=<=  OutDataTypeStr=boolean
  Constant1 : Constant  Value=CcCDP_BusbarTempRngFltLowThrd_C
  Logical Operator1 : Logic  AllPortsSameDT=off  OutDataTypeStr=boolean
  LbCDP_BusbarTempRngLowFlt_flg : Outport
  GbCDP_BusbarTempRngLowFlt_flg : Outport  Port=2
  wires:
  LbCDP_BusbarTempRngLowChk_flg/1 -> Logical Operator1/1
  Comparison3/1 -> Logical Operator1/2
  CDP_GbCDP_ChrgMaxCellVoltFltLv1_flg/1 -> GbCDP_BusbarTempRngLowFlt_flg/1  "GbCDP_BusbarTempRngLowFlt_flg"
  Logical Operator1/1 -> LbCDP_BusbarTempRngLowFlt_flg/1, CDP_GbCDP_ChrgMaxCellVoltFltLv1_flg/1  "LbCDP_BusbarTempRngLowFlt_flg"
  Constant1/1 -> Comparison3/2
  GcCDP_MinBusbarTemp_C/1 -> Comparison3/1

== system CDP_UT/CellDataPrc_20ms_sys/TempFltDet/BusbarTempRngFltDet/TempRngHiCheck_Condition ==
  LbCDP_AnyBusbarTempVld_flg : Inport
  Constant : Constant  Value=ASWTYPE_TRUE
  Constant1 : Constant  Value=CbCDP_MaxBusbarTempStateCheck_flg
  Constant2 : Constant  Value=ASWTYPE_TRUE
  Logical Operator : Logic  AllPortsSameDT=off  OutDataTypeStr=boolean
  Relational Operator : RelationalOperator  Operator===  OutDataTypeStr=boolean
  Relational Operator1 : RelationalOperator  Operator===  OutDataTypeStr=boolean
  LbCDP_BusbarTempRngHiChk_flg : Outport
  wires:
  LbCDP_AnyBusbarTempVld_flg/1 -> Relational Operator/1
  Constant/1 -> Relational Operator/2
  Relational Operator1/1 -> Logical Operator/2
  Constant2/1 -> Relational Operator1/2
  Relational Operator/1 -> Logical Operator/1
  Logical Operator/1 -> LbCDP_BusbarTempRngHiChk_flg/1  "LbCDP_BusbarTempRngHiChk_flg"
  Constant1/1 -> Relational Operator1/1

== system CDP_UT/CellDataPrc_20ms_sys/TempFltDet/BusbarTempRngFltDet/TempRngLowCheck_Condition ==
  LbCDP_AnyBusbarTempVld_flg : Inport
  Constant : Constant  Value=ASWTYPE_TRUE
  Constant3 : Constant  Value=CbCDP_MinBusbarTempStateCheck_flg
  Constant4 : Constant  Value=ASWTYPE_TRUE
  Logical Operator : Logic  AllPortsSameDT=off  OutDataTypeStr=boolean
  Relational Operator : RelationalOperator  Operator===  OutDataTypeStr=boolean
  Relational Operator2 : RelationalOperator  Operator===  OutDataTypeStr=boolean
  LbCDP_BusbarTempRngLowChk_flg : Outport
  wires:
  Logical Operator/1 -> LbCDP_BusbarTempRngLowChk_flg/1  "LbCDP_BusbarTempRngLowChk_flg"
  Relational Operator/1 -> Logical Operator/1
  Constant/1 -> Relational Operator/2
  LbCDP_AnyBusbarTempVld_flg/1 -> Relational Operator/1
  Constant4/1 -> Relational Operator2/2
  Constant3/1 -> Relational Operator2/1
  Relational Operator2/1 -> Logical Operator/2

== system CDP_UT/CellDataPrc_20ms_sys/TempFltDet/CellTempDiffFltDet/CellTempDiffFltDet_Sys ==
  LbCDP_DiffTempCheckCondition_flg : Inport
  GcCDP_MaxCellTemp_C : Inport  Port=2
  GcCDP_MinCellTemp_C : Inport  Port=3
  LbCDP_CellTempRngHiFlt_flg : Inport  Port=4
  LbCDP_CellTempRngLowFlt_flg : Inport  Port=5
  Add : Sum  Inputs=+-  OutDataTypeStr=Inherit: Inherit via back propagation
  Bus Creator : BusCreator  Inputs=4
  Bus Selector : BusSelector  OutputSignals=LcCDP_DiffCellTemp_C,LbCDP_CellTempRngHiFlt_flg,LbCDP_CellTempRngLowFlt_flg,LbCDP_DiffTempCheckCondition_flg
  Bus Selector1 : BusSelector  OutputSignals=LbCDP_DiffTempCheckCondition_flg,LcCDP_DiffCellTemp_C,LbCDP_CellTempRngHiFlt_flg,LbCDP_CellTempRngLowFlt_flg
  CellTempDiffFltLv1Det : Subsystem
  CellTempDiffFltLv2Det : Subsystem
  GbCDP_CellTempDiffFltLv2_flg : Outport
  GbCDP_CellTempDiffFltLv1_flg : Outport  Port=2
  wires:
  Add/1 -> Bus Creator/1  "LcCDP_DiffCellTemp_C"
  GcCDP_MaxCellTemp_C/1 -> Add/1
  GcCDP_MinCellTemp_C/1 -> Add/2
  Bus Creator/1 -> Bus Selector1/1, Bus Selector/1
  LbCDP_CellTempRngHiFlt_flg/1 -> Bus Creator/2
  LbCDP_CellTempRngLowFlt_flg/1 -> Bus Creator/3
  Bus Selector/1 -> CellTempDiffFltLv2Det/1(LcCDP_DiffCellTemp_C)  "<LcCDP_DiffCellTemp_C>"
  Bus Selector/2 -> CellTempDiffFltLv2Det/2(LbCDP_CellTempRngHiFlt_flg)  "<LbCDP_CellTempRngHiFlt_flg>"
  Bus Selector/3 -> CellTempDiffFltLv2Det/3(LbCDP_CellTempRngLowFlt_flg)  "<LbCDP_CellTempRngLowFlt_flg>"
  CellTempDiffFltLv2Det/1(GbCDP_CellTempDiffFltLv2_flg) -> GbCDP_CellTempDiffFltLv2_flg/1
  CellTempDiffFltLv1Det/1(GbCDP_CellTempDiffFltLv1_flg) -> GbCDP_CellTempDiffFltLv1_flg/1
  LbCDP_DiffTempCheckCondition_flg/1 -> Bus Creator/4
  Bus Selector/4 -> CellTempDiffFltLv2Det/4(LbCDP_DiffTempCheckCondition_flg)  "<LbCDP_DiffTempCheckCondition_flg>"
  Bus Selector1/1 -> CellTempDiffFltLv1Det/1(LbCDP_DiffTempCheckCondition_flg)  "<LbCDP_DiffTempCheckCondition_flg>"
  Bus Selector1/2 -> CellTempDiffFltLv1Det/2(LcCDP_DiffCellTemp_C)  "<LcCDP_DiffCellTemp_C>"
  Bus Selector1/3 -> CellTempDiffFltLv1Det/3(LbCDP_CellTempRngHiFlt_flg)  "<LbCDP_CellTempRngHiFlt_flg>"
  Bus Selector1/4 -> CellTempDiffFltLv1Det/4(LbCDP_CellTempRngLowFlt_flg)  "<LbCDP_CellTempRngLowFlt_flg>"

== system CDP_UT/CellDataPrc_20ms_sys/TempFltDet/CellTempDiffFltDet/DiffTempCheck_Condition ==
  LbCDP_AnyCellTempVld_flg : Inport
  Constant : Constant  Value=ASWTYPE_TRUE
  Constant1 : Constant  Value=CbCDP_DiffCellTempStateCheck_flg
  Constant2 : Constant  Value=ASWTYPE_TRUE
  Logical Operator : Logic  AllPortsSameDT=off  OutDataTypeStr=boolean
  Relational Operator : RelationalOperator  Operator===  OutDataTypeStr=boolean
  Relational Operator1 : RelationalOperator  Operator===  OutDataTypeStr=boolean
  LbCDP_DiffTempCheckCondition_flg : Outport
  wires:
  Constant1/1 -> Relational Operator1/1
  LbCDP_AnyCellTempVld_flg/1 -> Relational Operator/1
  Logical Operator/1 -> LbCDP_DiffTempCheckCondition_flg/1  "LbCDP_DiffTempCheckCondition_flg"
  Relational Operator1/1 -> Logical Operator/2
  Relational Operator/1 -> Logical Operator/1
  Constant/1 -> Relational Operator/2
  Constant2/1 -> Relational Operator1/2

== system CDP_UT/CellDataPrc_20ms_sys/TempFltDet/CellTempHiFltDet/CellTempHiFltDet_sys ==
  LbCDP_MaxTempCheckCondition_flg : Inport
  GcCDP_MaxCellTemp_C : Inport  Port=2
  Bus Creator : BusCreator  Inputs=2
  Bus Selector : BusSelector  OutputSignals=LbCDP_MaxTempCheckCondition_flg,GcCDP_MaxCellTemp_C
  Bus Selector1 : BusSelector  OutputSignals=LbCDP_MaxTempCheckCondition_flg,GcCDP_MaxCellTemp_C
  Bus Selector2 : BusSelector  OutputSignals=LbCDP_MaxTempCheckCondition_flg,GcCDP_MaxCellTemp_C
  CellTempHiFltLv1Det : Subsystem
  CellTempHiFltLv2Det : Subsystem
  CellTempHiFltLv3Det : Subsystem
  GbCDP_CellTempHiFltLv3_flg : Outport
  GbCDP_CellTempHiFltLv2_flg : Outport  Port=2
  GbCDP_CellTempHiFltLv1_flg : Outport  Port=3
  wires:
  GcCDP_MaxCellTemp_C/1 -> Bus Creator/1
  Bus Creator/1 -> Bus Selector2/1, Bus Selector1/1, Bus Selector/1
  CellTempHiFltLv3Det/1(GbCDP_CellTempHiFltLv3_flg) -> GbCDP_CellTempHiFltLv3_flg/1
  CellTempHiFltLv2Det/1(GbCDP_CellTempHiFltLv2_flg) -> GbCDP_CellTempHiFltLv2_flg/1
  CellTempHiFltLv1Det/1(GbCDP_CellTempHiFltLv1_flg) -> GbCDP_CellTempHiFltLv1_flg/1
  LbCDP_MaxTempCheckCondition_flg/1 -> Bus Creator/2
  Bus Selector/1 -> CellTempHiFltLv3Det/1(LbCDP_MaxTempCheckCondition_flg)  "<LbCDP_MaxTempCheckCondition_flg>"
  Bus Selector/2 -> CellTempHiFltLv3Det/2(GcCDP_MaxCellTemp_C)  "<GcCDP_MaxCellTemp_C>"
  Bus Selector1/1 -> CellTempHiFltLv2Det/1(LbCDP_MaxTempCheckCondition_flg)  "<LbCDP_MaxTempCheckCondition_flg>"
  Bus Selector1/2 -> CellTempHiFltLv2Det/2(GcCDP_MaxCellTemp_C)  "<GcCDP_MaxCellTemp_C>"
  Bus Selector2/1 -> CellTempHiFltLv1Det/1(LbCDP_MaxTempCheckCondition_flg)  "<LbCDP_MaxTempCheckCondition_flg>"
  Bus Selector2/2 -> CellTempHiFltLv1Det/2(GcCDP_MaxCellTemp_C)  "<GcCDP_MaxCellTemp_C>"

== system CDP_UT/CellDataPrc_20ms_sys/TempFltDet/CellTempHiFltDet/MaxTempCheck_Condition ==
  GbCDP_AllCellTempVld_flg : Inport
  LbCDP_AnyCellTempVld_flg : Inport  Port=2
  LbCDP_ChrgWkUp_flg : Inport  Port=3
  Constant : Constant  Value=ASWTYPE_TRUE
  Constant1 : Constant  Value=CbCDP_MaxCellTempStateCheck_flg
  Constant2 : Constant  Value=ASWTYPE_TRUE
  Constant3 : Constant  Value=ASWTYPE_TRUE
  Constant4 : Constant  Value=ASWTYPE_FALSE
  Logical Operator : Logic  Inputs=3  AllPortsSameDT=off  OutDataTypeStr=boolean
  Relational Operator{,1..3} (4 alike) : RelationalOperator  Operator===  OutDataTypeStr=boolean
  Terminator : Terminator
  LbCDP_MaxTempCheckCondition_flg : Outport
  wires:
  Constant1/1 -> Relational Operator1/1
  Logical Operator/1 -> LbCDP_MaxTempCheckCondition_flg/1  "LbCDP_MaxTempCheckCondition_flg"
  Relational Operator/1 -> Terminator/1
  Constant2/1 -> Relational Operator1/2
  Relational Operator1/1 -> Logical Operator/2
  Constant/1 -> Relational Operator/2
  GbCDP_AllCellTempVld_flg/1 -> Relational Operator/1
  Constant3/1 -> Relational Operator2/2
  Relational Operator2/1 -> Logical Operator/1
  LbCDP_AnyCellTempVld_flg/1 -> Relational Operator2/1
  LbCDP_ChrgWkUp_flg/1 -> Relational Operator3/1
  Constant4/1 -> Relational Operator3/2
  Relational Operator3/1 -> Logical Operator/3

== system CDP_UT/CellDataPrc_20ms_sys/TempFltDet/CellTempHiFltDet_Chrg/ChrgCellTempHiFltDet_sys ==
  LbCDP_ChrgMaxTempChkCond_flg : Inport
  GcCDP_MaxCellTemp_C : Inport  Port=2
  Bus Creator : BusCreator  Inputs=2
  Bus Selector : BusSelector  OutputSignals=LbCDP_ChrgMaxTempChkCond_flg,GcCDP_MaxCellTemp_C
  Bus Selector1 : BusSelector  OutputSignals=LbCDP_ChrgMaxTempChkCond_flg,GcCDP_MaxCellTemp_C
  Bus Selector2 : BusSelector  OutputSignals=LbCDP_ChrgMaxTempChkCond_flg,GcCDP_MaxCellTemp_C
  CellTempHiFltLv1Det_Chrg : Subsystem
  CellTempHiFltLv2Det_Chrg : Subsystem
  CellTempHiFltLv3Det_Chrg : Subsystem
  GbCDP_ChrgCellTempHiFltLv3_flg : Outport
  GbCDP_ChrgCellTempHiFltLv2_flg : Outport  Port=2
  GbCDP_ChrgCellTempHiFltLv1_flg : Outport  Port=3
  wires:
  Bus Selector2/2 -> CellTempHiFltLv1Det_Chrg/2(GcCDP_MaxCellTemp_C)  "<GcCDP_MaxCellTemp_C>"
  Bus Selector2/1 -> CellTempHiFltLv1Det_Chrg/1(LbCDP_ChrgMaxTempChkCond_flg)  "<LbCDP_ChrgMaxTempChkCond_flg>"
  Bus Selector1/2 -> CellTempHiFltLv2Det_Chrg/2(GcCDP_MaxCellTemp_C)  "<GcCDP_MaxCellTemp_C>"
  Bus Selector1/1 -> CellTempHiFltLv2Det_Chrg/1(LbCDP_ChrgMaxTempChkCond_flg)  "<LbCDP_ChrgMaxTempChkCond_flg>"
  Bus Selector/2 -> CellTempHiFltLv3Det_Chrg/2(GcCDP_MaxCellTemp_C)  "<GcCDP_MaxCellTemp_C>"
  Bus Selector/1 -> CellTempHiFltLv3Det_Chrg/1(LbCDP_ChrgMaxTempChkCond_flg)  "<LbCDP_ChrgMaxTempChkCond_flg>"
  LbCDP_ChrgMaxTempChkCond_flg/1 -> Bus Creator/2
  CellTempHiFltLv1Det_Chrg/1(GbCDP_ChrgCellTempHiFltLv1_flg) -> GbCDP_ChrgCellTempHiFltLv1_flg/1
  CellTempHiFltLv2Det_Chrg/1(GbCDP_ChrgCellTempHiFltLv2_flg) -> GbCDP_ChrgCellTempHiFltLv2_flg/1
  CellTempHiFltLv3Det_Chrg/1(GbCDP_ChrgCellTempHiFltLv3_flg) -> GbCDP_ChrgCellTempHiFltLv3_flg/1
  Bus Creator/1 -> Bus Selector/1, Bus Selector1/1, Bus Selector2/1
  GcCDP_MaxCellTemp_C/1 -> Bus Creator/1

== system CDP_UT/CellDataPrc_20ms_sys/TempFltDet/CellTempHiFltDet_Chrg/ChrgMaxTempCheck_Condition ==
  GbCDP_AllCellTempVld_flg : Inport
  LbCDP_AnyCellTempVld_flg : Inport  Port=2
  LbCDP_ChrgWkUp_flg : Inport  Port=3
  Constant{,2..4} (4 alike) : Constant  Value=ASWTYPE_TRUE
  Constant1 : Constant  Value=CbCDP_MaxCellTempStateCheck_flg
  Logical Operator : Logic  Inputs=3  AllPortsSameDT=off  OutDataTypeStr=boolean
  Relational Operator{,1..3} (4 alike) : RelationalOperator  Operator===  OutDataTypeStr=boolean
  Terminator : Terminator
  LbCDP_ChrgMaxTempChkCond_flg : Outport
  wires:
  Relational Operator3/1 -> Logical Operator/3
  Constant4/1 -> Relational Operator3/2
  LbCDP_ChrgWkUp_flg/1 -> Relational Operator3/1
  LbCDP_AnyCellTempVld_flg/1 -> Relational Operator2/1
  Relational Operator2/1 -> Logical Operator/1
  Constant3/1 -> Relational Operator2/2
  GbCDP_AllCellTempVld_flg/1 -> Relational Operator/1
  Constant/1 -> Relational Operator/2
  Relational Operator1/1 -> Logical Operator/2
  Constant2/1 -> Relational Operator1/2
  Relational Operator/1 -> Terminator/1
  Logical Operator/1 -> LbCDP_ChrgMaxTempChkCond_flg/1  "LbCDP_ChrgMaxTempChkCond_flg"
  Constant1/1 -> Relational Operator1/1

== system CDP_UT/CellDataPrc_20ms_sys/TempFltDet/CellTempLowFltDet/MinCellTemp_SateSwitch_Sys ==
  LbCDP_MinTempCheckCondition_flg : Inport
  GcCDP_MinCellTemp_C : Inport  Port=2
  Bus Creator : BusCreator  Inputs=2
  Bus Selector : BusSelector  OutputSignals=GcCDP_MinCellTemp_C,LbCDP_MinTempCheckCondition_flg
  Bus Selector1 : BusSelector  OutputSignals=GcCDP_MinCellTemp_C,LbCDP_MinTempCheckCondition_flg
  Bus Selector2 : BusSelector  OutputSignals=GcCDP_MinCellTemp_C,LbCDP_MinTempCheckCondition_flg
  CellTempLowFltLv1Det : Subsystem
  CellTempLowFltLv2Det : Subsystem
  CellTempLowFltLv3Det : Subsystem
  GbCDP_CellTempLowFltLv3_flg : Outport
  GbCDP_CellTempLowFltLv2_flg : Outport  Port=2
  GbCDP_CellTempLowFltLv1_flg : Outport  Port=3
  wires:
  GcCDP_MinCellTemp_C/1 -> Bus Creator/2
  Bus Creator/1 -> Bus Selector2/1, Bus Selector1/1, Bus Selector/1
  Bus Selector1/1 -> CellTempLowFltLv2Det/1(GcCDP_MinCellTemp_C)  "<GcCDP_MinCellTemp_C>"
  Bus Selector1/2 -> CellTempLowFltLv2Det/2(LbCDP_MinTempCheckCondition_flg)  "<LbCDP_MinTempCheckCondition_flg>"
  CellTempLowFltLv3Det/1(GbCDP_CellTempLowFltLv3_flg) -> GbCDP_CellTempLowFltLv3_flg/1
  Bus Selector2/2 -> CellTempLowFltLv1Det/2(LbCDP_MinTempCheckCondition_flg)  "<LbCDP_MinTempCheckCondition_flg>"
  CellTempLowFltLv2Det/1(GbCDP_CellTempLowFltLv2_flg) -> GbCDP_CellTempLowFltLv2_flg/1
  CellTempLowFltLv1Det/1(GbCDP_CellTempLowFltLv1_flg) -> GbCDP_CellTempLowFltLv1_flg/1
  LbCDP_MinTempCheckCondition_flg/1 -> Bus Creator/1
  Bus Selector/1 -> CellTempLowFltLv3Det/1(GcCDP_MinCellTemp_C)  "<GcCDP_MinCellTemp_C>"
  Bus Selector/2 -> CellTempLowFltLv3Det/2(LbCDP_MinTempCheckCondition_flg)  "<LbCDP_MinTempCheckCondition_flg>"
  Bus Selector2/1 -> CellTempLowFltLv1Det/1(GcCDP_MinCellTemp_C)  "<GcCDP_MinCellTemp_C>"

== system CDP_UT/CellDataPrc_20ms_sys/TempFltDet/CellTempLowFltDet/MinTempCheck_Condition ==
  GbCDP_AllCellTempVld_flg : Inport
  LbCDP_AnyCellTempVld_flg : Inport  Port=2
  LbCDP_ChrgWkUp_flg : Inport  Port=3
  Constant : Constant  Value=ASWTYPE_TRUE
  Constant1 : Constant  Value=CbCDP_MinCellTempStateCheck_flg
  Constant2 : Constant  Value=ASWTYPE_TRUE
  Constant3 : Constant  Value=ASWTYPE_TRUE
  Constant4 : Constant  Value=ASWTYPE_FALSE
  Logical Operator : Logic  Inputs=3  AllPortsSameDT=off  OutDataTypeStr=boolean
  Relational Operator{,1..3} (4 alike) : RelationalOperator  Operator===  OutDataTypeStr=boolean
  Terminator : Terminator
  LbCDP_MinTempCheckCondition_flg : Outport
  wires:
  Relational Operator1/1 -> Logical Operator/2
  GbCDP_AllCellTempVld_flg/1 -> Relational Operator/1
  Constant1/1 -> Relational Operator1/1
  Constant2/1 -> Relational Operator1/2
  Logical Operator/1 -> LbCDP_MinTempCheckCondition_flg/1  "LbCDP_MinTempCheckCondition_flg"
  Constant/1 -> Relational Operator/2
  Relational Operator/1 -> Terminator/1
  LbCDP_AnyCellTempVld_flg/1 -> Relational Operator2/1
  Constant3/1 -> Relational Operator2/2
  Relational Operator2/1 -> Logical Operator/1
  LbCDP_ChrgWkUp_flg/1 -> Relational Operator3/1
  Constant4/1 -> Relational Operator3/2
  Relational Operator3/1 -> Logical Operator/3

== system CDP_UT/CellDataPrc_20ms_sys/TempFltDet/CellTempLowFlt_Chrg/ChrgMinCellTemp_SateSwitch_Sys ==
  LbCDP_ChrgMinTempChkCond_flg : Inport
  GcCDP_MinCellTemp_C : Inport  Port=2
  Bus Creator : BusCreator  Inputs=2
  Bus Selector : BusSelector  OutputSignals=GcCDP_MinCellTemp_C,LbCDP_ChrgMinTempChkCond_flg
  Bus Selector1 : BusSelector  OutputSignals=GcCDP_MinCellTemp_C,LbCDP_ChrgMinTempChkCond_flg
  Bus Selector2 : BusSelector  OutputSignals=GcCDP_MinCellTemp_C,LbCDP_ChrgMinTempChkCond_flg
  CellTempLowFltLv1Det_Chrg : Subsystem
  CellTempLowFltLv2Det_Chrg : Subsystem
  CellTempLowFltLv3Det_Chrg : Subsystem
  GbCDP_ChrgCellTempLowFltLv3_flg : Outport
  GbCDP_ChrgCellTempLowFltLv2_flg : Outport  Port=2
  GbCDP_ChrgCellTempLowFltLv1_flg : Outport  Port=3
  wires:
  Bus Selector2/1 -> CellTempLowFltLv1Det_Chrg/1(GcCDP_MinCellTemp_C)  "<GcCDP_MinCellTemp_C>"
  Bus Selector/2 -> CellTempLowFltLv3Det_Chrg/2(LbCDP_ChrgMinTempChkCond_flg)  "<LbCDP_ChrgMinTempChkCond_flg>"
  Bus Selector/1 -> CellTempLowFltLv3Det_Chrg/1(GcCDP_MinCellTemp_C)  "<GcCDP_MinCellTemp_C>"
  LbCDP_ChrgMinTempChkCond_flg/1 -> Bus Creator/1
  CellTempLowFltLv1Det_Chrg/1(GbCDP_ChrgCellTempLowFltLv1_flg) -> GbCDP_ChrgCellTempLowFltLv1_flg/1
  CellTempLowFltLv2Det_Chrg/1(GbCDP_ChrgCellTempLowFltLv2_flg) -> GbCDP_ChrgCellTempLowFltLv2_flg/1
  Bus Selector2/2 -> CellTempLowFltLv1Det_Chrg/2(LbCDP_ChrgMinTempChkCond_flg)  "<LbCDP_ChrgMinTempChkCond_flg>"
  CellTempLowFltLv3Det_Chrg/1(GbCDP_ChrgCellTempLowFltLv3_flg) -> GbCDP_ChrgCellTempLowFltLv3_flg/1
  Bus Selector1/2 -> CellTempLowFltLv2Det_Chrg/2(LbCDP_ChrgMinTempChkCond_flg)  "<LbCDP_ChrgMinTempChkCond_flg>"
  Bus Selector1/1 -> CellTempLowFltLv2Det_Chrg/1(GcCDP_MinCellTemp_C)  "<GcCDP_MinCellTemp_C>"
  Bus Creator/1 -> Bus Selector/1, Bus Selector1/1, Bus Selector2/1
  GcCDP_MinCellTemp_C/1 -> Bus Creator/2

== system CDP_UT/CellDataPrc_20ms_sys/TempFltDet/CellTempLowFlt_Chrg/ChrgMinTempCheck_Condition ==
  GbCDP_AllCellTempVld_flg : Inport
  LbCDP_AnyCellTempVld_flg : Inport  Port=2
  LbCDP_ChrgWkUp_flg : Inport  Port=3
  Constant{,2..4} (4 alike) : Constant  Value=ASWTYPE_TRUE
  Constant1 : Constant  Value=CbCDP_MinCellTempStateCheck_flg
  Logical Operator : Logic  Inputs=3  AllPortsSameDT=off  OutDataTypeStr=boolean
  Relational Operator{,1..3} (4 alike) : RelationalOperator  Operator===  OutDataTypeStr=boolean
  Terminator : Terminator
  LbCDP_ChrgMinTempChkCond_flg : Outport
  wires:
  Relational Operator3/1 -> Logical Operator/3
  Constant4/1 -> Relational Operator3/2
  LbCDP_ChrgWkUp_flg/1 -> Relational Operator3/1
  Relational Operator2/1 -> Logical Operator/1
  Constant3/1 -> Relational Operator2/2
  LbCDP_AnyCellTempVld_flg/1 -> Relational Operator2/1
  Relational Operator/1 -> Terminator/1
  Constant/1 -> Relational Operator/2
  Logical Operator/1 -> LbCDP_ChrgMinTempChkCond_flg/1  "LbCDP_ChrgMinTempChkCond_flg"
  Constant2/1 -> Relational Operator1/2
  Constant1/1 -> Relational Operator1/1
  GbCDP_AllCellTempVld_flg/1 -> Relational Operator/1
  Relational Operator1/1 -> Logical Operator/2
